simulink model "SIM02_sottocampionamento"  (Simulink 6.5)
settings: Solver=ode1  StartTime=0.0  StopTime=10  FixedStep=0.0001  RelTol=1e-3

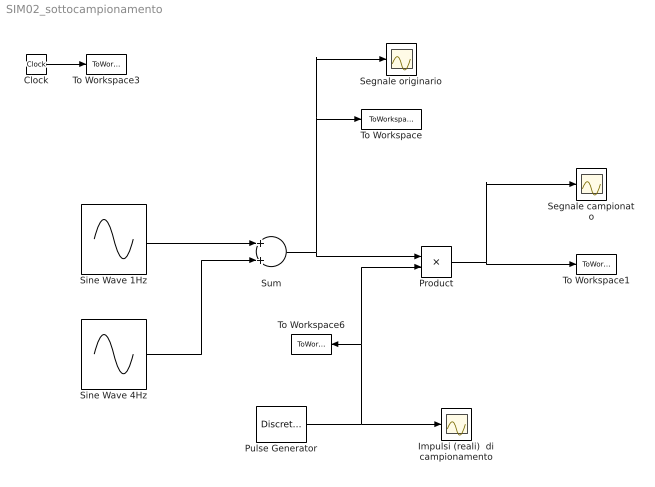
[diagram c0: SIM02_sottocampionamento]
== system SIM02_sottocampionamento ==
  Clock : Clock
  Impulsi (reali)  di campionamento : Scope
  Product : Product
  Pulse Generator : DiscretePulseGenerator  PulseType=Time based  Period=0.15  PulseWidth=2/3  SampleTime=0.02
  Segnale campionato : Scope
  Segnale originario : Scope
  Sine Wave 1Hz : Sin  Frequency=2*pi  SampleTime=0
  Sine Wave 4Hz : Sin  Amplitude=0.5  Frequency=8*pi  SampleTime=0
  Sum : Sum
  To Workspace : ToWorkspace  VariableName=x  SampleTime=-1  SaveFormat=Array
  To Workspace1 : ToWorkspace  VariableName=xs  SampleTime=-1  SaveFormat=Array
  To Workspace3 : ToWorkspace  VariableName=tempo  SampleTime=-1  SaveFormat=Array
  To Workspace6 : ToWorkspace  VariableName=samp  SampleTime=-1  SaveFormat=Array
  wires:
  Sine Wave 1Hz/1 -> Sum/1
  Sine Wave 4Hz/1 -> Sum/2
  Sum/1 -> To Workspace/1, Segnale originario/1, Product/1
  Product/1 -> To Workspace1/1, Segnale campionato/1
  Pulse Generator/1 -> Product/2, To Workspace6/1, Impulsi (reali)  di campionamento/1
  Clock/1 -> To Workspace3/1
